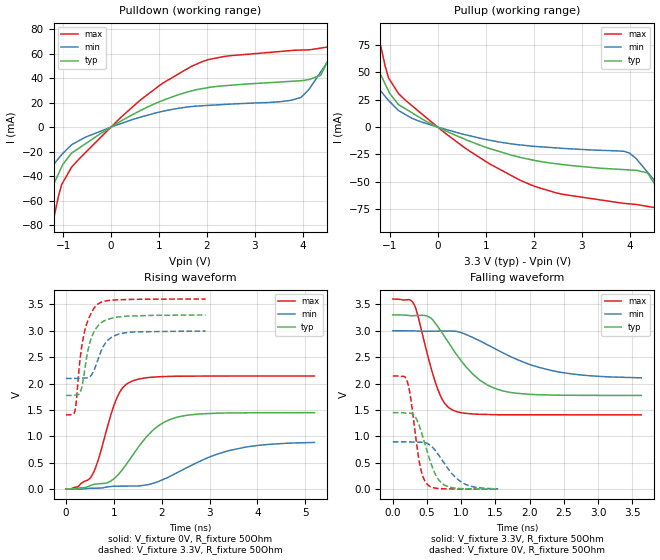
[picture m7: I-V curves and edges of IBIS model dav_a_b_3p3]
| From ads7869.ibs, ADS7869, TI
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|   dav_a_b_3p3 Model
[Model]   dav_a_b_3p3
Model_type   Output
Polarity   Non-Inverting
Vmeas = 1.65
Vref = 1.65
Cref = 30pF
Rref = 50
|   typ   min   max
|   (nom PVT)   (fast PVT)   (slow PVT)
|C_comp from frequency sweep method (F=8MHz)
|C_comp   3.647e-12   3.528e-12   3.770e-12
|ON state : BUFFER OUTPUT TURNED HIGH
|C_comp   3.647e-12   3.528e-12   3.770e-12
|OFF state: BUFFER OUTPUT TURNED LOW
|C_comp   3.303e-12   3.111e-12   3.332e-12
|C_comp from LC tank measurement(L=1nH)
|Resonant Frequency(Hz)   3.130e+09   3.140e+09   3.130e+09
C_comp   2.502e-12   2.494e-12   2.532e-12
|ON state : BUFFER OUTPUT TURNED HIGH
|Resonant Frequency(Hz)   3.130e+09   3.140e+09   3.130e+09
|C_comp   2.588e-12   2.572e-12   2.588e-12
|OFF state: BUFFER OUTPUT TURNED LOW
|Resonant Frequency(Hz)   3.240e+09   3.240e+09   3.200e+09
|C_comp   2.415e-12   2.415e-12   2.476e-12
| Where nom  PVT is Nominal Process, 3.3V, 36C
|   Fast PVT is Strong Process,  3.6V, -40C
|   Slow PVT is Weak Process,   3V, 96C
[Voltage Range]   3.3   3   3.6
|Ambient Temperature   25   85   -40
|Junction Temperature
[Temperature Range]   36   96   -40
[Pullup Reference]   3.3   3   3.6
[Pulldown Reference]   0   0   0
[Power Clamp Reference]   3.3   3   3.6
[GND Clamp Reference]   0   0   0
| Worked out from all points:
|   slope of the pulldown table from 0 to 0.495 V, typ, clamps not added: 44.4 ohm
|   slope of the pullup table from 0 to 0.495 V, typ, clamps not added: 50.3 ohm
|   falling waveform, V_fixture 3.3V, R_fixture 50Ohm: 20-80 % time 556ps typ, 947ps min, 282ps max; typ from 3.3 V to 1.77 V
|   rising waveform, V_fixture 0V, R_fixture 50Ohm: 20-80 % time 770ps typ, 1.31ns min, 430ps max; typ from 0 V to 1.45 V
|   rising waveform, V_fixture 3.3V, R_fixture 50Ohm: 20-80 % time 234ps typ, 271ps min, 211ps max; typ from 1.77 V to 3.3 V
|   falling waveform, V_fixture 0V, R_fixture 50Ohm: 20-80 % time 222ps typ, 322ps min, 138ps max; typ from 1.45 V to 0.002 V
[Pulldown]
|   Voltage   I(typ)   I(min)   I(max)
-3.3V     -255.2mA   -141.4mA   -538.1mA
-1.383V   -64.61mA   -39.8mA    -116mA
-1.264V   -52.78mA   -33.79mA   -89.82mA
-1.032V   -32.59mA   -22.5mA    -46.99mA
-679.2mV  -17.41mA   -11.28mA   -26.48mA
1.916V    31.54mA    17.5mA     53.71mA
3.96V     37.92mA    24.24mA    62.93mA
4.372V    42.45mA    45.15mA    64.53mA
4.66V     67.43mA    61.93mA    66.32mA
4.793V    81.59mA    69.71mA    80.13mA
5.052V    109.1mA    84.85mA    136mA
6.6V      273.7mA    175.3mA    495.8mA
[Pullup]
|   Voltage   I(typ)   I(min)   I(max)
-3.3V     272.5mA    157mA      562.7mA
-1.407V   70.22mA    45.07mA    123.7mA
-1.274V   56.01mA    37.57mA    92.83mA
-1.032V   33.21mA    24.43mA    45.18mA
-823.2mV  20.64mA    15.24mA    30.71mA
638.4mV   -12.48mA   -7.628mA   -21.28mA
1.916V    -29.54mA   -17.18mA   -52.39mA
3.996V    -39.13mA   -23.74mA   -70.11mA
4.372V    -41.89mA   -41.3mA    -72.47mA
4.825V    -81.16mA   -65mA      -89.06mA
5.056V    -103.9mA   -77.06mA   -135.6mA
6.6V      -256.6mA   -157.9mA   -476.2mA
[Ramp]
R_load = 50
|   typ   min   max
dV/dt_r   0.869326/7.70131e-10   0.535502/1.31856e-09   1.28577/4.30156e-10
dV/dt_f   0.914951/5.56222e-10   0.541879/9.65541e-10   1.31593/2.81676e-10
[Falling Waveform]
V_fixture = 3.3V
V_fixture_min = 3V
V_fixture_max = 3.6V
R_fixture = 50Ohm
|   Time   V(typ)   V(min)   V(max)
0s        3.3V       3V         3.6V
316.5ps   3.287V     2.997V     3.484V
504.4ps   3.276V     2.99V      2.559V
655.5ps   3.083V     2.992V     1.899V
747ps     2.908V     2.994V     1.648V
864.1ps   2.679V     2.994V     1.506V
1.272ns   2.064V     2.809V     1.418V
1.6ns     1.864V     2.589V     1.409V
2.432ns   1.78V      2.219V     1.409V
3.632ns   1.775V     2.108V     1.408V
[Rising Waveform]
V_fixture = 0V
V_fixture_min = 0V
V_fixture_max = 0V
R_fixture = 50Ohm
|   Time   V(typ)   V(min)   V(max)
0s        781.6pV    11.3nV     670.9pV
538.2ps   78.79mV    17mV       250.6mV
673.2ps   101.3mV    19.65mV    550.3mV
1.061ns   245.5mV    56.13mV    1.722V
1.207ns   403.5mV    57.77mV    1.941V
1.388ns   633.7mV    59.8mV     2.049V
1.851ns   1.142V     119.6mV    2.123V
2.319ns   1.362V     310.6mV    2.139V
3.392ns   1.443V     727.2mV    2.143V
5.192ns   1.448V     884.9mV    2.143V
[Rising Waveform]
V_fixture = 3.3V
V_fixture_min = 3V
V_fixture_max = 3.6V
R_fixture = 50Ohm
|   Time   V(typ)   V(min)   V(max)
0s        1.775V     2.097V     1.407V
177.7ps   1.779V     2.097V     1.448V
212.7ps   1.781V     2.097V     1.632V
291.6ps   1.823V     2.101V     2.435V
421.1ps   2.43V      2.104V     3.095V
524.6ps   2.846V     2.153V     3.327V
655.5ps   3.075V     2.418V     3.498V
832.8ps   3.2V       2.777V     3.564V
1.076ns   3.259V     2.927V     3.585V
2.919ns   3.299V     2.992V     3.6V
[Falling Waveform]
V_fixture = 0V
V_fixture_min = 0V
V_fixture_max = 0V
R_fixture = 50Ohm
|   Time   V(typ)   V(min)   V(max)
0s        1.449V     895.5mV    2.143V
212.7ps   1.441V     897mV      2.036V
259.5ps   1.439V     894.9mV    1.736V
307.4ps   1.404V     891.5mV    1.269V
399.5ps   1.15V      888.9mV    433.8mV
510.8ps   677.4mV    862.3mV    82.16mV
635.4ps   249mV      707.6mV    17.96mV
773ps     66.23mV    450.2mV    7.046mV
1.076ns   7.689mV    85mV       1.812mV
1.539ns   1.647mV    8.296mV    821.1uV
